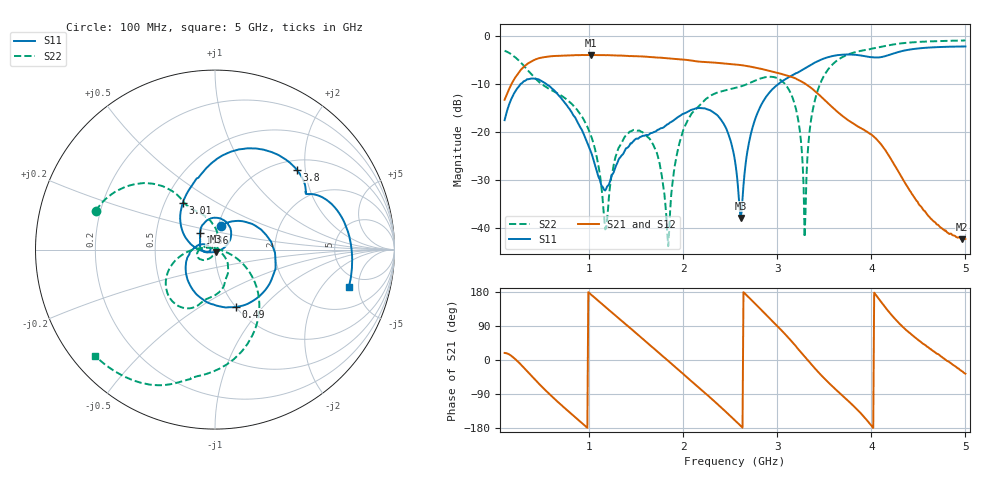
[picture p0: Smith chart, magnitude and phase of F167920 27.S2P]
!  2-Port S-parameters saved by WinCal
! VAR MeasName=S-Parameters (CALIBRATED_DATA) read from VNA (N5242A)
! VAR MeasDate=2016-11-22 9:56:30
! VAR NAME=F167920 27
! VAR FILENAME=F167920 27.S2P
! VAR DATE=2016-11-22 9:56:30
! VAR PHYS_PORTS=1,2
# Hz S DB R 50
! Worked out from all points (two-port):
!   491 points, 100 MHz to 5 GHz, reference 50 ohm
!   highest |S21| = -3.99 dB at 1.02 GHz (marker M1); lowest = -42.2 dB at 4.96 GHz (marker M2)
!   |S21| within 3 dB of the highest: 277.1 MHz to 2.851 GHz (2.574 GHz wide, 165 % of centre)
!   lowest |S11| = -37.8 dB at 2.61 GHz (marker M3), VSWR 1.03, Z = 50.3 - j1.24 ohm
!   |S11| at or under -10 dB: start of sweep to 271.4 MHz; 541.3 MHz to 3.013 GHz (2.472 GHz wide, 139 % of centre)
!   |S22| runs from -43.7 to -1.0 dB; largest |S21 - S12| = 0.0012
!   S11 on the Smith chart (normalised r, x): 100 MHz: 1.03, +0.27; 490 MHz: 1.00, -0.73; 1.86 GHz: 0.83, +0.16; 3.01 GHz: 0.62, +0.35; 3.8 GHz: 1.20, +1.80; 5 GHz: 3.73, -3.85
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1e8  -17.53 76.2  -13.29 18.6  -13.29 18.6  -3.12 162.0
4.9e8  -9.36 -69.8  -4.55 -69.0  -4.55 -68.9  -9.97 123.5
9.2e8  -19.49 170.5  -4.00 -166.0  -3.99 -166.0  -16.77 95.7
1.02e9  -24.22 151.3  -3.99 172.5  -3.99 172.5  -20.83 81.2
1.17e9  -32.14 178.5  -4.04 140.5  -4.04 140.5  -40.21 -11.8
1.4e9  -23.32 -175.5  -4.18 91.6  -4.18 91.7  -20.59 -143.6
1.74e9  -19.46 141.4  -4.54 19.1  -4.54 19.1  -25.88 159.9
1.83e9  -18.40 134.3  -4.68 -0.2  -4.68 -0.2  -41.07 94.7
1.86e9  -18.00 131.9  -4.73 -6.6  -4.74 -6.7  -36.48 3.0
2.04e9  -15.86 110.9  -5.04 -45.9  -5.04 -45.9  -17.83 -55.2
2.37e9  -16.67 54.2  -5.63 -117.8  -5.64 -117.8  -11.74 -91.8
2.55e9  -26.01 10.2  -5.95 -159.3  -5.96 -159.3  -10.88 -101.6
2.61e9  -37.85 -74.6  -6.09 -173.7  -6.09 -173.7  -10.54 -103.5
2.75e9  -18.19 170.9  -6.55 152.2  -6.56 152.1  -9.42 -109.2
3.01e9  -10.05 125.0  -7.76 87.3  -7.78 87.3  -8.90 -137.8
3.2e9  -7.77 104.6  -8.92 35.8  -8.93 35.7  -15.32 -172.9
3.29e9  -6.81 96.1  -9.88 9.1  -9.89 9.1  -41.82 127.1
3.37e9  -5.88 88.4  -11.00 -13.9  -11.02 -13.9  -16.12 -24.9
3.8e9  -3.92 44.5  -18.16 -118.7  -18.18 -118.6  -3.56 -87.8
4.19e9  -3.98 29.1  -25.00 125.9  -25.05 126.3  -1.97 -109.3
4.96e9  -2.24 -13.6  -42.25 -29.3  -42.21 -28.6  -1.00 -137.4
5e9  -2.23 -15.5  -42.20 -36.2  -42.23 -36.7  -0.98 -138.4
